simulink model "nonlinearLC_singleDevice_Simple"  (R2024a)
settings: Solver=ode45  StartTime=0.0  StopTime=tstop  MaxStep=tstep  RelTol=1e-3  EnableMultiTasking=on
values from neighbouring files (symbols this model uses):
  Clin = [Cper Cpqr]    [CallNlinC_singleDevice_Simple.m]
  Cx = interp1(Vtest,Ctest,vx,'linear')    [CallNlinC_singleDevice_Simple.m]
  Il0 = 0.5    [CallNlinC_singleDevice_Simple.m]
  Ll = 12.5e-6    (= 1.25e-05)    [CallNlinC_singleDevice_Simple.m]
  Vc0 = 0    [CallNlinC_singleDevice_Simple.m]
  Vg = 100    [CallNlinC_singleDevice_Simple.m]
  vlin = [min(vx)-.1 max(vx)+.1]    [CallNlinC_singleDevice_Simple.m]
  Vout = -Vg    (= -100)    [CallNlinC_singleDevice_Simple.m]
  vx = 0.01:.01:Vg+25    [CallNlinC_singleDevice_Simple.m]

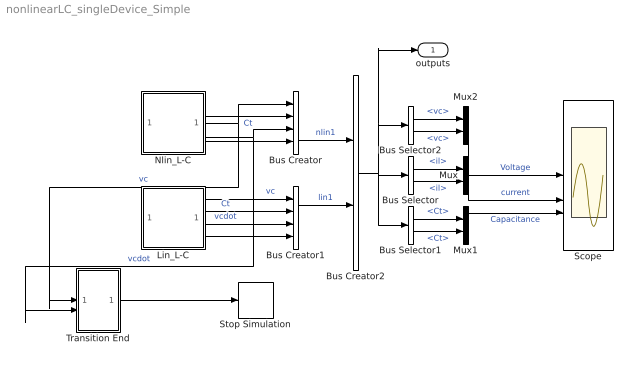
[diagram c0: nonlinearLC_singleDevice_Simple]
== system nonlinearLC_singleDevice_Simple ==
  Bus Creator : BusCreator  Inputs=4
  Bus Creator1 : BusCreator  Inputs=4
  Bus Creator2 : BusCreator  Inputs=2
  Bus Selector : BusSelector  OutputSignals=nlin1.il,lin1.il
  Bus Selector1 : BusSelector  OutputSignals=nlin1.Ct,lin1.Ct
  Bus Selector2 : BusSelector  OutputSignals=nlin1.vc,lin1.vc
  Lin_L-C : Subsystem  mask{Cx=Clin, vx=vlin, Ll=Ll, Vg=Vg, Vout=Vout, Vc0=Vc0, Il0=Il0}
      mask prompts: Cx "Capacitance Curve"; vx "Voltage Curve"; Ll "Inductance"; Vg "Clamped/Target Voltage"; Vout "DC Voltage in Res. Circuit"; Vc0 "Initial Cap voltage"; Il0 "Initial Inductor Current"
  Mux : Mux  Inputs=2
  Mux1 : Mux  Inputs=2
  Mux2 : Mux  Inputs=2
  Nlin_L-C : Subsystem  mask{Cx=Cx, vx=vx, Ll=Ll, Vg=Vg, Vout=Vout, Vc0=Vc0, Il0=Il0}
      mask prompts: Cx "Capacitance Curve"; vx "Voltage Curve"; Ll "Inductance"; Vg "Clamped/Target Voltage"; Vout "DC Voltage in Res. Circuit"; Vc0 "Initial Cap voltage"; Il0 "Initial Inductor Current"
  Scope : Scope  NumInputPorts=3
  Stop Simulation : Stop
  Transition End : Subsystem
  outputs : Outport
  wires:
  Transition End/1(STOP) -> Stop Simulation/1
  Nlin_L-C/1(vc) -> Transition End/1(Vc), Bus Creator/1  "vc"
  Nlin_L-C/3(vcdot) -> Transition End/2(Vcdot), Bus Creator/3  "vcdot"
  Nlin_L-C/4(il) -> Bus Creator/4  "il"
  Nlin_L-C/2(Ct) -> Bus Creator/2  "Ct"
  Lin_L-C/1(vc) -> Bus Creator1/1  "vc"
  Lin_L-C/3(vcdot) -> Bus Creator1/3  "vcdot"
  Lin_L-C/4(il) -> Bus Creator1/4  "il"
  Lin_L-C/2(Ct) -> Bus Creator1/2  "Ct"
  Bus Creator/1 -> Bus Creator2/1  "nlin1"
  Bus Creator1/1 -> Bus Creator2/2  "lin1"
  Bus Creator2/1 -> Bus Selector/1, Bus Selector1/1, Bus Selector2/1, outputs/1
  Bus Selector/2 -> Mux/2  "<il>"
  Bus Selector/1 -> Mux/1  "<il>"
  Bus Selector1/2 -> Mux1/2  "<Ct>"
  Bus Selector1/1 -> Mux1/1  "<Ct>"
  Bus Selector2/2 -> Mux2/2  "<vc>"
  Bus Selector2/1 -> Mux2/1  "<vc>"
  Mux2/1 -> Scope/1  "Voltage"
  Mux/1 -> Scope/2  "current"
  Mux1/1 -> Scope/3  "Capacitance"

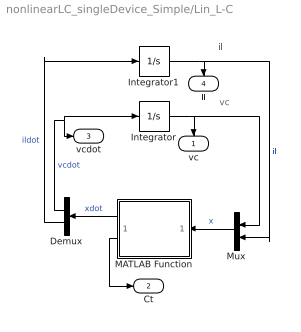
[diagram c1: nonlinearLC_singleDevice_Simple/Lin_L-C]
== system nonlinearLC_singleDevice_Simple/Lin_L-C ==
  note: il
  note: vc
  Demux : Demux  Outputs=2
  Integrator : Integrator  InitialCondition=Vc0
  Integrator1 : Integrator  InitialCondition=Il0
  MATLAB Function : MATLAB Function  TreatAsAtomicUnit=on
  Mux : Mux  Inputs=2
  vc : Outport
  Ct : Outport  Port=2
  vcdot : Outport  Port=3
  il : Outport  Port=4
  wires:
  Mux/1 -> MATLAB Function/1(x)  "x"
  MATLAB Function/1(xdot) -> Demux/1  "xdot"
  Demux/1 -> Integrator/1, vcdot/1  "vcdot"
  Integrator/1 -> Mux/1, vc/1
  Demux/2 -> Integrator1/1  "ildot"
  Integrator1/1 -> Mux/2, il/1  "il"
  MATLAB Function/2(Cpout) -> Ct/1

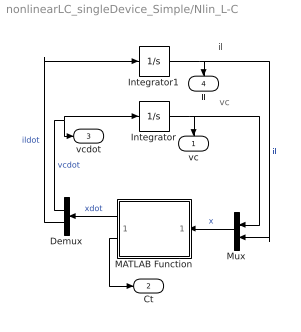
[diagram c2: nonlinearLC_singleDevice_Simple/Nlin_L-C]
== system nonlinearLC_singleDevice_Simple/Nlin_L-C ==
  note: il
  note: vc
  Demux : Demux  Outputs=2
  Integrator : Integrator  InitialCondition=Vc0
  Integrator1 : Integrator  InitialCondition=Il0
  MATLAB Function : MATLAB Function  TreatAsAtomicUnit=on
  Mux : Mux  Inputs=2
  vc : Outport
  Ct : Outport  Port=2
  vcdot : Outport  Port=3
  il : Outport  Port=4
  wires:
  Mux/1 -> MATLAB Function/1(x)  "x"
  MATLAB Function/1(xdot) -> Demux/1  "xdot"
  Demux/1 -> Integrator/1, vcdot/1  "vcdot"
  Integrator/1 -> Mux/1, vc/1
  Demux/2 -> Integrator1/1  "ildot"
  Integrator1/1 -> Mux/2, il/1  "il"
  MATLAB Function/2(Cpout) -> Ct/1

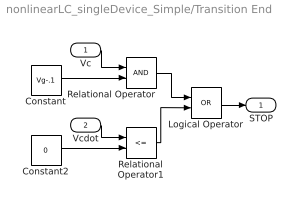
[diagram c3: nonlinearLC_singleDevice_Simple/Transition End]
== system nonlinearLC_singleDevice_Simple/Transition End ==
  Vc : Inport
  Vcdot : Inport  Port=2
  Constant : Constant  Value=Vg-.1
  Constant2 : Constant  Value=0
  Logical Operator : Logic  Operator=OR  AllPortsSameDT=off  OutDataTypeStr=boolean
  Relational Operator : RelationalOperator  OutDataTypeStr=boolean
  Relational Operator1 : RelationalOperator  Operator=<=  OutDataTypeStr=boolean
  STOP : Outport
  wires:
  Relational Operator/1 -> Logical Operator/1
  Relational Operator1/1 -> Logical Operator/2
  Constant/1 -> Relational Operator/2
  Constant2/1 -> Relational Operator1/2
  Vc/1 -> Relational Operator/1
  Logical Operator/1 -> STOP/1
  Vcdot/1 -> Relational Operator1/1

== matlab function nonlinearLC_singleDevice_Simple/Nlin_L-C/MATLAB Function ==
function [xdot,Cpout]= fcn(x, Cx, vx, Vg, Ll, Vout)

vc = x(1);

%% Find and output instantaneous Capacitance
index = find(vc < vx, 1);
Cp = Cx(index);
Cpout = Cp(1);


%% Calculate States 
% x = [vcp il]

A = [0      1/Cp;
     -1/Ll  0];
B = [0;     1/Ll]; 

if(x(1) < Vg)
    xdot = A*x + B*Vout;
else
     xdot = 0*x;
end

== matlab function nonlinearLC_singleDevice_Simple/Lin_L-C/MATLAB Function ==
function [xdot,Cpout]= fcn(x, Cx, vx, Vg, Ll, Vout)
%#codegen

vc = x(1);

%% Find and output instantaneous Capacitance
index = find(vc < vx, 1);
Cp = Cx(index);
Cpout = Cp(1);


%% Calculate States 
% x = [vcp il]

A = [0      1/Cp;
     -1/Ll  0];
B = [0;     1/Ll]; 

if(x(1) < Vg)
    xdot = A*x + B*Vout;
else
     xdot = 0*x;
end
%  xdot(1) = -400/10e-9;
